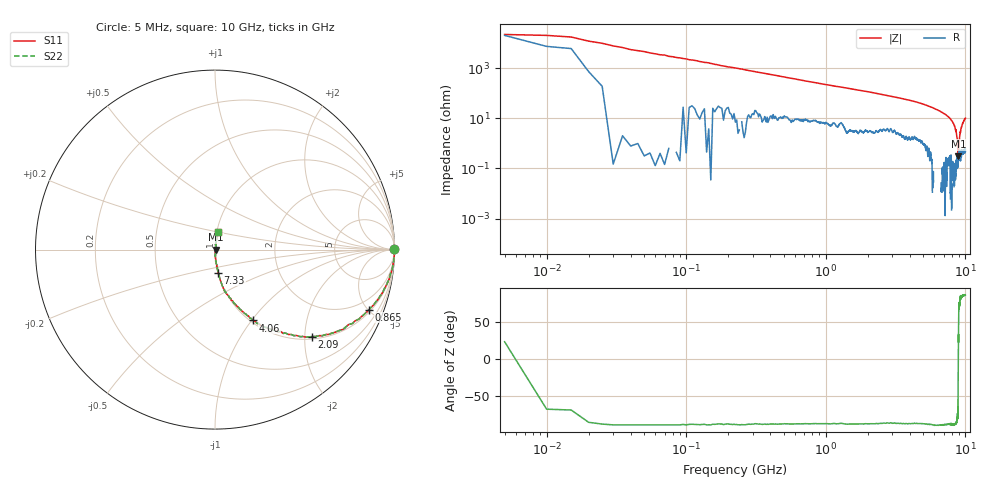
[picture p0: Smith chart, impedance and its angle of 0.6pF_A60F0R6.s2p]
! Amotech Co.,Ltd.
! http://www.amotech.co.kr/
! Part Number: A60F0R6
! These Parameters are Measured in Series Mode Connection
! Operation Temp=25[degC], DC Bias Voltage=0[V]
! Freq. Start=5[MHz] Stop=10[GHz], 2000[Steps]
! Date: Monday, July 20, 2020, 03:11:53
# GHZ S RI R 50.000000
!Freq.(Hz) S11(Real) S11(Imag) S21(Real) S21(Imag) S12(Real) S12(Imag) S22(Real) S22(Imag)
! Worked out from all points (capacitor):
!   2000 points, 5 MHz to 10 GHz, reference 50 ohm
!   read as one part in series: C = 707 fF near 55 MHz
!   lowest |Z| = 306 mohm at 8.9 GHz (marker M1)
!   series resonance near 8.904 GHz, so ESL is about 450 pH
!   S11 on the Smith chart (normalised r, x): 5 MHz: open; 865 MHz: 1.14, -5.08; 2.09 GHz: 1.06, -2.17; 4.06 GHz: 1.03, -1.01; 7.33 GHz: 1.00, -0.26; 10 GHz: 1.01, +0.20
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0.005  0.9958 0.0018  0.00422 -0.0018  0.00422 -0.0018  0.9958 0.0018
0.09  0.9984 -0.0395  0.00157 0.0395  0.00157 0.0395  0.9984 -0.0395
0.225  0.9895 -0.0984  0.0105 0.0984  0.0105 0.0984  0.9895 -0.0984
0.495  0.9472 -0.2125  0.0528 0.2125  0.0528 0.2125  0.9472 -0.2125
0.865  0.8589 -0.3343  0.1411 0.3343  0.1411 0.3343  0.8589 -0.3343
1.675  0.6442 -0.4688  0.3558 0.4688  0.3558 0.4688  0.6442 -0.4688
2.09  0.5405 -0.4843  0.4595 0.4843  0.4595 0.4843  0.5405 -0.4843
3.34  0.2995 -0.4402  0.7005 0.4402  0.7005 0.4402  0.2995 -0.4402
4.06  0.2113 -0.3946  0.7887 0.3946  0.7887 0.3946  0.2113 -0.3946
5.005  0.1209 -0.3139  0.8791 0.3139  0.8791 0.3139  0.1209 -0.3139
6.67  0.032 -0.1768  0.968 0.1768  0.968 0.1768  0.032 -0.1768
7.33  0.0172 -0.1286  0.9828 0.1286  0.9828 0.1286  0.0172 -0.1286
8.03  0.00647 -0.0777  0.9935 0.0777  0.9935 0.0777  0.00647 -0.0777
8.335  0.0023 -0.0489  0.9977 0.0489  0.9977 0.0489  0.0023 -0.0489
8.61  0.00252 -0.028  0.9975 0.028  0.9975 0.028  0.00252 -0.028
8.735  0.00293 -0.0148  0.9971 0.0148  0.9971 0.0148  0.00293 -0.0148
8.86  0.0018 -0.0037  0.9982 0.0037  0.9982 0.0037  0.0018 -0.0037
8.9  0.00295 -0.000803  0.9971 0.000803  0.9971 0.000803  0.00295 -0.000803
9.025  0.00359 0.0109  0.9964 -0.0109  0.9964 -0.0109  0.00359 0.0109
9.17  0.00533 0.0256  0.9947 -0.0256  0.9947 -0.0256  0.00533 0.0256
9.51  0.00797 0.0565  0.992 -0.0565  0.992 -0.0565  0.00797 0.0565
10  0.0156 0.0986  0.9844 -0.0986  0.9844 -0.0986  0.0156 0.0986
